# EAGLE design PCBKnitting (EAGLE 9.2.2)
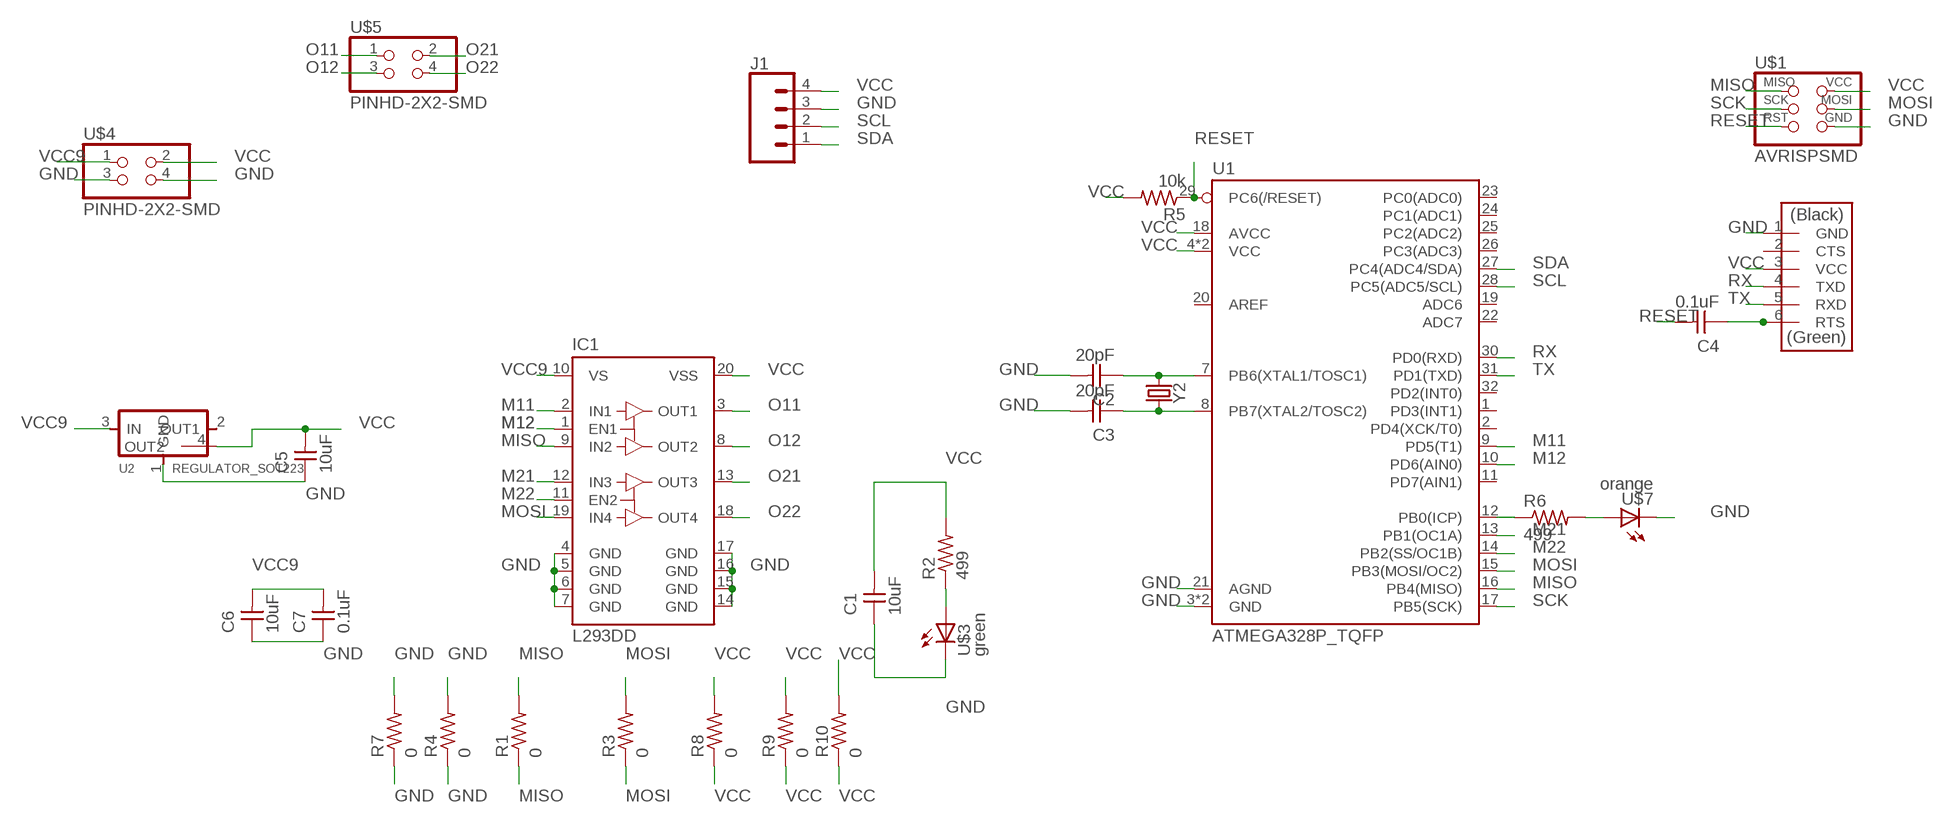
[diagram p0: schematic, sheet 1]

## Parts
C1  10uF  CAP-UNPOLARIZEDFAB  [C1206FAB]
C2  20pF  CAP-UNPOLARIZEDFAB  [C1206FAB]
C3  20pF  CAP-UNPOLARIZEDFAB  [C1206FAB]
C4  0.1uF  CAP-UNPOLARIZEDFAB  [C1206FAB]
C5  10uF  CAP-UNPOLARIZEDFAB  [C1206FAB]
C6  10uF  CAP-UNPOLARIZEDFAB  [C1206FAB]
C7  0.1uF  CAP-UNPOLARIZEDFAB  [C1206FAB]
IC1  L293DD  [SO20]
J1  CONN_04SMD_RA_FEMALE  [1X04_SMD_RA_FEMALE]
R1  0  RES-US1206FAB  [R1206FAB]
R2  499  RES-US1206FAB  [R1206FAB]
R3  0  RES-US1206FAB  [R1206FAB]
R4  0  RES-US1206FAB  [R1206FAB]
R5  10k  RES-US1206FAB  [R1206FAB]
R6  499  RES-US1206FAB  [R1206FAB]
R7  0  RES-US1206FAB  [R1206FAB]
R8  0  RES-US1206FAB  [R1206FAB]
R9  0  RES-US1206FAB  [R1206FAB]
R10  0  RES-US1206FAB  [R1206FAB]
U1  ATMEGA328P_TQFP  [TQFP32-08]
U2  REGULATOR_SOT223  [SOT223]
U$1  AVRISPSMD  [2X03SMD]
U$2  FTDI-SMD-HEADER  [1X06SMD]
U$3  green  LEDFAB1206  [LED1206FAB]
U$4  PINHD-2X2-SMD  [2X02SMD]
U$5  PINHD-2X2-SMD  [2X02SMD]
U$7  orange  LEDFAB1206  [LED1206FAB]
Y2  CRYSTALSMD-HC49UP  [HC49UP]

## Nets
GND: C1.1 C2.2 C3.2 C5.1 C6.1 C7.1 IC1.4(GND) IC1.5(GND) IC1.6(GND) IC1.7(GND) IC1.14(GND) IC1.15(GND) IC1.16(GND) IC1.17(GND) J1.3 R4.1 R4.2 R7.1 R7.2 U1.3(GND) U1.5(GND) U1.21(AGND) U2.1(GND) U$1.6(GND) U$2.1(GND) U$3.2(C) U$4.3 U$4.4 U$7.2(C)
M11: IC1.2(IN1) U1.9(PD5(T1))
M12: IC1.1(EN1) U1.10(PD6(AIN0))
M21: IC1.12(IN3) U1.13(PB1(OC1A))
M22: IC1.11(EN2) U1.14(PB2(SS/OC1B))
MISO: IC1.9(IN2) R1.1 R1.2 U1.16(PB4(MISO)) U$1.1(MISO)
MOSI: IC1.19(IN4) R3.1 R3.2 U1.15(PB3(MOSI/OC2)) U$1.4(MOSI)
N$1: R2.1 U$3.1(A)
N$4: C2.1 U1.7(PB6(XTAL1/TOSC1)) Y2.1
N$5: C3.1 U1.8(PB7(XTAL2/TOSC2)) Y2.2
N$8: R6.1 U1.12(PB0(ICP))
N$9: R6.2 U$7.1(A)
N$14: C4.1 U$2.6(RTS)
O11: IC1.3(OUT1) U$5.1
O12: IC1.8(OUT2) U$5.3
O21: IC1.13(OUT3) U$5.2
O22: IC1.18(OUT4) U$5.4
RESET: C4.2 R5.1 U1.29(PC6(/RESET)) U$1.5(RST)
RX: U1.30(PD0(RXD)) U$2.4(TXD)
SCK: U1.17(PB5(SCK)) U$1.3(SCK)
SCL: J1.2 U1.28(PC5(ADC5/SCL))
SDA: J1.1 U1.27(PC4(ADC4/SDA))
TX: U1.31(PD1(TXD)) U$2.5(RXD)
VCC: C1.2 C5.2 IC1.20(VSS) J1.4 R2.2 R5.2 R8.1 R8.2 R9.1 R9.2 R10.1 R10.2 U1.4(VCC) U1.6(VCC) U1.18(AVCC) U2.4(OUT2) U$1.2(VCC) U$2.3(VCC) U$4.2
VCC9: C6.2 C7.2 IC1.10(VS) U2.3(IN) U$4.1
Unconnected: U1.1(PD3(INT1)) U1.2(PD4(XCK/T0)) U1.11(PD7(AIN1)) U1.19(ADC6) U1.20(AREF) U1.22(ADC7) U1.23(PC0(ADC0)) U1.24(PC1(ADC1)) U1.25(PC2(ADC2)) U1.26(PC3(ADC3)) U1.32(PD2(INT0)) U2.2(OUT1) U$2.2(CTS)

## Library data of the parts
C1-C7 = fab:CAP-UNPOLARIZED
IC1 = st-microelectronics:L293DD: PUSH-PULL FOUR CHANNEL DRIVER WITH DIODES Source: http://www.st.com/stonline/books/pdf/docs/1330.pdf; OC_FARNELL: unknown
J1 = SparkFun-Connectors:CONN_04: Multi connection point. Often used as Generic Header-pin footprint for 0.1 inch spaced/style header connections On any of the 0.1 inch spaced packages, you can populate with these: Break Away Headers - Straight (PRT-00116) Break Away Male Headers - Right Angle (PRT-00553) Female Headers (PRT-00115)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; PROD_ID: CONN-12382; SPICEPREFIX: E
R1-R10 = fab:RES-US: Resistor (US Symbol)
U1 = SparkFun-IC-Microcontroller:ATMEGA328P_TQFP: Popular 328P in QFP Storefront component: ATmega328 - TQFP (COM-13448) Datasheet SparkFun Products SparkFun RedBoard - Programmed with Arduino (DEV-12757) Arduino Pro Mini 328 - 5V/16MHz (DEV-11113) Arduino Pro Mini 328 - 3.3V/8MHz (DEV-11114) SparkFun OpenLog (DEV-13712) SparkFun MicroView - OLED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; PROD_ID: IC-09069
U2 = fab:REGULATOR_SOT223
U$1 = fab:AVRISP
U$2 = fab:FTDI-SMD-HEADER
U$3 U$7 = fab:LED: LED
U$4 U$5 = fab:PINHD-2X2-SMD
Y2 = SparkFun-Clocks:CRYSTAL: Crystals (Generic)

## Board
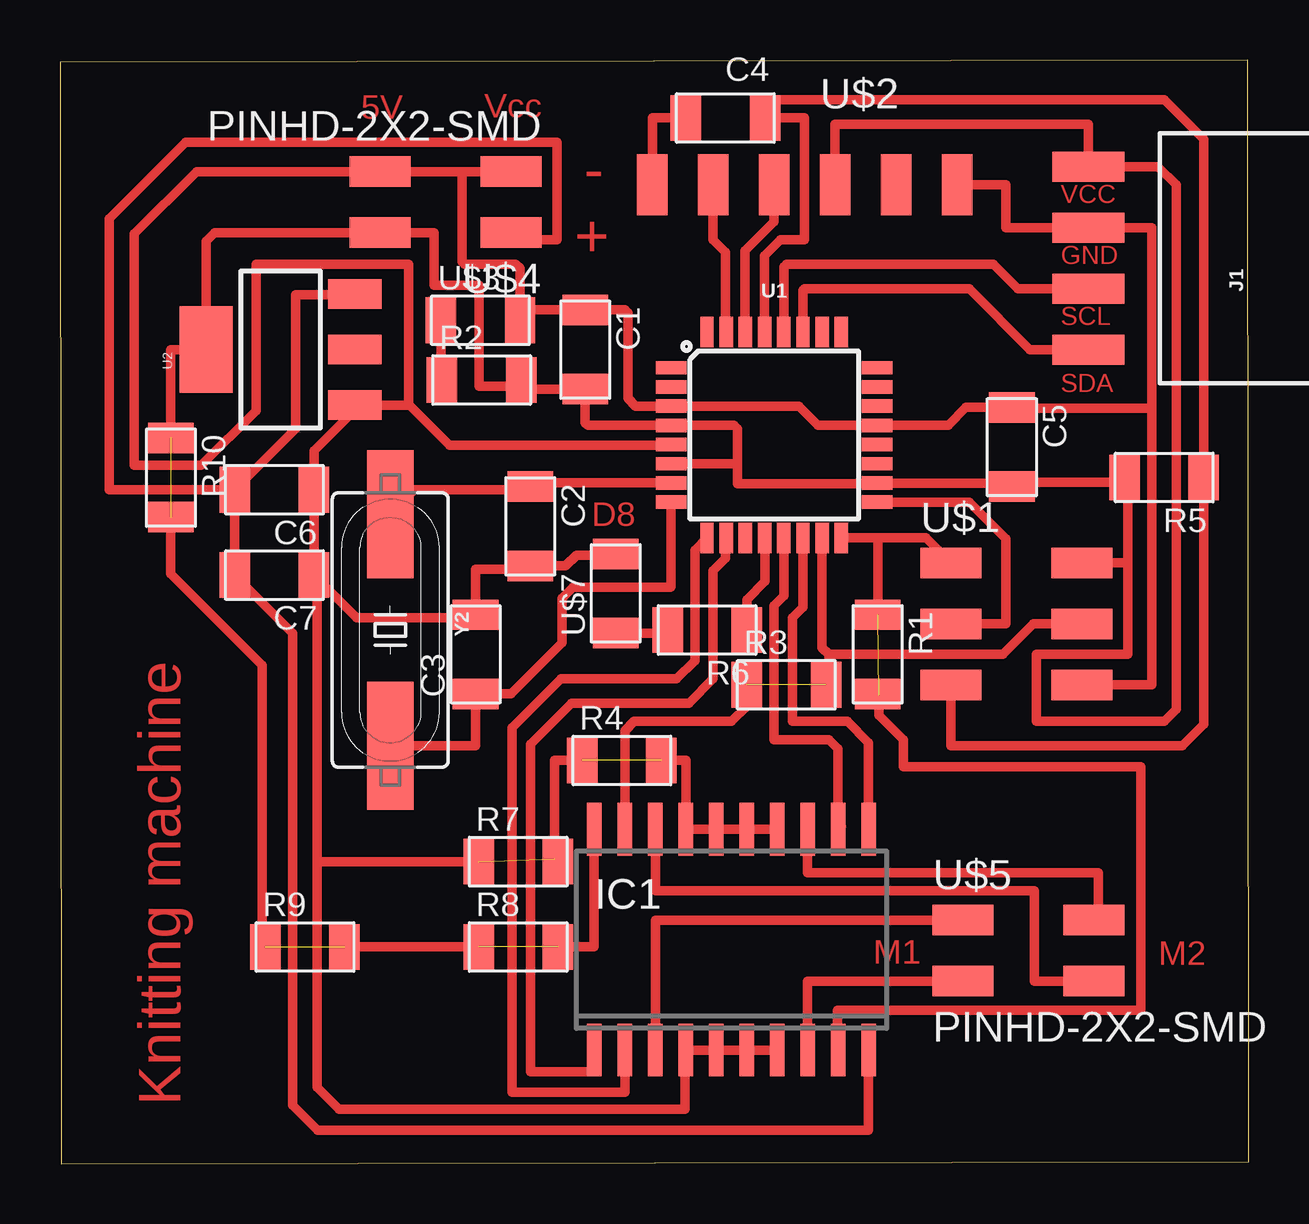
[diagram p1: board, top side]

Size 49.56 x 46 mm. Coordinates in mm from the lower left corner, seen from the top.
Outline: 0.05,0 49.56,0.1 49.51,46 0,45.9 0.05,0
Copper layers (1*16): Top 0.035mm / dielectric 1.5mm / Bottom 0.035mm
Design rules "default *": minimum track width 0.4mm, minimum drill 0.35mm, track to track 0.3mm, track to pad 0.3mm, pad to pad 0.3mm, via to via 0.3mm, smd to smd 0.3mm, copper to edge 40mil, drill to drill 6mil, minimum pad ring 10mil, minimum via ring 8mil, stop-mask expansion 4mil, vias tented up to drill 0mil, thermal gap 10mil

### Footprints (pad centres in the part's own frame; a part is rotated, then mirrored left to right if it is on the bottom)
C1206FAB = smd 1.27 x 1.905: 1 -1.651,0; 2 1.651,0
SO20 = smd 0.6 x 2.2: 1 -5.715,-4.6; 2 -4.445,-4.6; 3 -3.175,-4.6; 4 -1.905,-4.6; 5 -0.635,-4.6; 6 0.635,-4.6; 7 1.905,-4.6; 8 3.175,-4.6; 9 4.445,-4.6; 10 5.715,-4.6; 11 5.715,4.6; 12 4.445,4.6; 13 3.175,4.6; 14 1.905,4.6; 15 0.635,4.6; 16 -0.635,4.6; 17 -1.905,4.6; 18 -3.175,4.6; 19 -4.445,4.6; 20 -5.715,4.6
1X04_SMD_RA_FEMALE = smd 1.25 x 3: 1 -3.81,7.225; 2 -1.27,7.225; 3 1.27,7.225; 4 3.81,7.225
R1206FAB = smd 1.27 x 1.905: 1 -1.651,0; 2 1.651,0
TQFP32-08 = smd 1.27 x 0.559: 1 -4.293,2.8; 2 -4.293,2; 3 -4.293,1.2; 4 -4.293,0.4; 5 -4.293,-0.4; 6 -4.293,-1.2; 7 -4.293,-2; 8 -4.293,-2.8; 17 4.293,-2.8; 18 4.293,-2; 19 4.293,-1.2; 20 4.293,-0.4; 21 4.293,0.4; 22 4.293,1.2; 23 4.293,2; 24 4.293,2.8 | smd 0.559 x 1.27: 9 -2.8,-4.293; 10 -2,-4.293; 11 -1.2,-4.293; 12 -0.4,-4.293; 13 0.4,-4.293; 14 1.2,-4.293; 15 2,-4.293; 16 2.8,-4.293; 25 2.8,4.293; 26 2,4.293; 27 1.2,4.293; 28 0.4,4.293; 29 -0.4,4.293; 30 -1.2,4.293; 31 -2,4.293; 32 -2.8,4.293
SOT223 = smd 1.219 x 2.235: 1 -2.311,-3.099; 2 0,-3.099; 3 2.311,-3.099 | smd 3.6 x 2.2: 4 0,3.099
2X03SMD = smd 2.54 x 1.27: 1 -2.54,2.54; 2 2.92,2.54; 3 -2.54,0; 4 2.92,0; 5 -2.54,-2.54; 6 2.92,-2.54
1X06SMD = smd 2.54 x 1.27: 1 0,6.35; 2 0,3.81; 3 0,1.27; 4 0,-1.27; 5 0,-3.81; 6 0,-6.35
LED1206FAB = smd 1.27 x 1.905: 1 -1.651,0; 2 1.651,0
2X02SMD = smd 2.54 x 1.27: 1 -2.54,1.27; 2 2.92,1.27; 3 -2.54,-1.27; 4 2.92,-1.27
HC49UP = smd 5.334 x 1.93: 1 -4.826,0; 2 4.826,0

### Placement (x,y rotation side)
C1  21.89,33.93 270 top
C2  19.61,26.57 270 top
C3  17.32,21.23 90 top
C4  27.74,43.59 0 top
C5  39.67,29.87 270 top
C6  8.94,28.09 180 top
C7  8.94,24.54 180 top
IC1  27.99,9.35 0 top
J1  50.09,37.74 90 top
R1  34.09,21.23 270 top
R2  17.58,32.66 0 top
R3  30.28,19.96 0 top
R4  23.42,16.81 0 top
R5  46.02,28.6 180 top
R6  26.97,22.25 180 top
R7  19.1,12.6 0 top
R8  19.1,9.04 0 top
R9  10.21,9.04 0 top
R10  4.62,28.6 270 top
U1  29.77,30.38 0 top
U2  9.19,33.93 90 top
U$1  39.67,22.5 0 top
U$2  31.04,40.79 270 top
U$3  17.53,35.15 0 top
U$4  16.26,40.08 180 top
U$5  40.18,8.89 0 top
U$7  23.16,23.77 90 top
Y2  13.77,22.25 270 top

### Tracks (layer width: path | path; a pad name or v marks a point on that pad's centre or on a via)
GND  (2 unrouted)
  Top 0.4: U$2.1 39.42,40.79 39.42,39.01 J1.3 | U1.5 25.5,29.96 16.24,29.96 14.58,31.62 | 43.74,39.01 J1.3 | U$1.6 45.52,19.96 45.52,31.5 | 22.66,35.59 23.55,35.59 23.67,35.46 23.67,31.9 24,31.58 U1.3 30.8,31.58 31.6,30.78 U1.21 37.03,30.78 37.77,31.52 C5.1 39.67,31.5 45.52,31.5 | 22.66,35.59 C1.1 19.61,35.59 U$3.2 | J1.3 45.52,39.01 45.52,31.5 | C3.2 16.94,23.27 | IC1.14 IC1.15 IC1.16 IC1.17 26.09,16.81 R4.2 | IC1.7 IC1.6 IC1.5 IC1.4 26.06,4.72 26.06,2.29 11.63,2.29 10.72,3.2 10.72,12.6 | 16.76,41.35 U$4.4 5.69,41.35 3.1,38.76 3.1,29.11 5.89,29.11 8.18,31.39 8.18,37.49 14.53,37.49 14.53,31.67 14.58,31.62 | 16.76,41.35 U$4.3 | C3.2 17.32,24.79 19.48,24.79 C2.2 21.08,24.92 21.54,25.37 22.81,25.37 22.86,25.43 U$7.2 | U$3.2 19.18,35.79 | 22.4,35.84 22.66,35.59 | U2.1 12.5,31.62 | 12.5,31.62 14.58,31.62 | 12.5,31.62 10.59,29.72 C6.1 C7.1 10.72,24.41 | 10.72,24.41 12.37,22.76 17.2,22.76 C3.2 | U$3.2 19.18,35.38 | R4.1 20.62,16.81 20.62,12.73 R7.2 | R7.1 10.72,12.6 | 10.72,12.6 10.72,24.41 | U$3.2 19.18,37.31 19,37.49 16.87,37.49 16.76,37.59 16.76,41.35
M11
  Top 0.4: U1.9 26.46,25.58 26.46,20.97 25.7,20.22 20.88,20.22 18.85,18.19 18.85,3 23.55,3 IC1.2
M12
  Top 0.4: U1.10 27.75,26.07 27.75,25.24 27.23,24.72 27.23,20.22 26.21,19.2 21.32,19.2 19.61,17.49 19.61,3.84 22.28,3.84 IC1.1
M21
  Top 0.4: 30.19,26.07 U1.13 30.17,23.67 29.77,23.27 29.77,17.68 32.05,17.68 32.44,17.3 IC1.12 32.56,14.07
M22
  Top 0.4: 30.99,26.07 U1.14 30.97,23.2 30.53,22.76 30.53,18.44 32.82,18.44 33.71,17.55 IC1.11
MISO  (1 unrouted)
  Top 0.4: 34.09,26.09 36.09,26.09 U$1.1 | 34.09,26.09 U1.16 | 34.09,26.09 R1.1 | R1.2 34.14,19.53 34.14,18.69 35.15,17.68 35.15,16.56 45.06,16.56 45.06,6.4 32.41,6.4 32.41,4.77 IC1.9
MOSI  (1 unrouted)
  Top 0.4: U$1.4 40.56,22.5 39.29,21.23 32.05,21.23 | U1.15 31.77,21.52 32.05,21.23 | IC1.19 23.55,18.06 23.93,18.44 27.99,18.44 28.63,19.08 R3.1 | R3.2 32.05,20.09 32.05,21.23
N$1
  Top 0.4: U$3.1 15.87,32.72 R2.1
N$4
  Top 0.4: Y2.1 14.78,28.09 19.48,28.09 C2.1 19.77,28.38 U1.7
N$5
  Top 0.4: U1.8 25.48,24.05 25.45,24.03 21.39,24.03 20.93,23.57 20.93,21.72 18.8,19.58 C3.1 | C3.1 17.45,19.71 | C3.1 17.32,17.42 Y2.2
N$8
  Top 0.4: U1.12 29.39,26.07 29.39,24.28 28.63,23.52 R6.1
N$9
  Top 0.4: R6.2 25.2,22.12 U$7.1
N$14
  Top 0.4: U$2.6 24.69,43.59 C4.1
O11
  Top 0.4: U$5.1 24.82,10.16 IC1.3
O12
  Top 0.4: U$5.3 31.17,7.62 IC1.8
O21
  Top 0.4: U$5.2 43.28,10.34 43.28,12.14 31.17,12.14 IC1.13
O22
  Top 0.4: U$5.4 40.61,7.62 40.61,11.38 24.82,11.38 IC1.18
RESET
  Top 0.4: U1.29 29.37,37.85 30.02,38.51 31.04,38.51 31.04,43.59 C4.2 29.51,43.71 29.51,44.35 46.02,44.35 47.68,42.7 R5.1 47.68,18.31 46.79,17.42 37.13,17.42 U$1.5
RX
  Top 0.4: 29.77,39.78 U$2.4 29.77,39.27 28.55,38.05 28.55,34.69 U1.30
SCK
  Top 0.4: 34.07,27.58 U1.17 37.9,27.58 39.42,26.06 39.42,22.5 U$1.3
SCL
  Top 0.4: U1.28 30.17,37.38 30.28,37.49 38.91,37.49 39.93,36.47 J1.2
SDA
  Top 0.4: 30.99,34.69 U1.27 30.97,36.4 31.04,36.47 37.9,36.47 40.44,33.93 J1.1
TX
  Top 0.4: U$2.5 27.23,38.51 27.75,37.99 27.75,34.69 U1.31
VCC  (3 unrouted)
  Top 0.4: U$2.3 32.31,43.33 42.86,43.33 J1.4 45.77,41.55 46.53,40.79 46.53,18.95 46.02,18.44 40.69,18.44 40.69,21.23 44.5,21.23 44.5,25.04 | U1.6 28.24,29.18 | 34.04,28.36 33.22,28.36 33.21,28.35 28.24,28.35 28.24,29.18 | 34.04,28.36 U1.18 34.08,28.36 | R5.2 44.12,28.85 | R2.2 19.42,32.47 | 19.42,32.47 19.61,32.28 C1.2 21.89,30.89 22,30.78 U1.4 28.1,30.78 28.24,30.63 28.24,29.18 | 44.18,28.41 43.99,28.22 | R5.2 44.5,28.47 44.5,25.04 | U$1.2 44.5,25.04 | R5.2 44.18,28.41 | 44.18,28.41 39.86,28.41 C5.2 39.54,28.36 34.04,28.36 | U$4.2 6.45,38.81 6.1,38.46 U2.4 4.62,33.93 R10.1 | U$4.2 13.44,38.91 | R8.2 22.25,9.04 22.25,13.92 IC1.20 | R8.1 R9.2 | R9.1 8.43,9.17 8.43,20.78 4.62,24.59 R10.2 | U$4.2 15.6,38.81 15.6,36.61 17.47,36.61 17.47,32.41 19.35,32.41 19.42,32.47
VCC9
  Top 0.4: U2.3 12.32,36.22 9.83,36.22 9.83,30.63 C6.2 | C6.2 C7.2 | C7.2 9.7,22.12 9.7,2.44 10.73,1.41 33.71,1.41 IC1.10 | C7.2 7.48,24.35 | U$4.1 19.1,38.51 20.73,38.51 20.73,42.57 5.23,42.57 2.06,39.4 2.06,28.09 C6.2

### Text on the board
Top: 5V | Vcc | - | VCC | + | GND | SCL | SDA | D8 | M1 | M2 | Knitting machine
